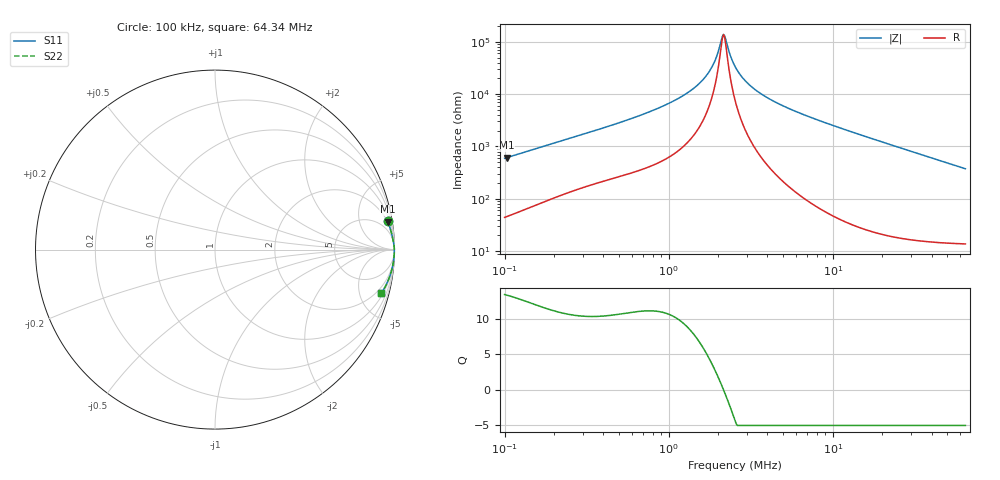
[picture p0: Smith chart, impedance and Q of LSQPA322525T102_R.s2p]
! LSQPA322525T102_R  S-PARAMETER MODEL  ( General Type )
! Model Generated by TAIYO YUDEN Corporation (http://www.ty-top.com)
! Version 1.0
! TAIYO YUDEN Control No. 111018NG25SB-FKC
! Copyright(c) 2011 TAIYO YUDEN CO.,LTD. All Rights Reserved.
! Product Description (link to TY-COMPAS)
! https://ds.yuden.co.jp/TYCOMPAS/or/detail?pn=LSQPA322525T102KR&u=M
! Products Name : Inductors
! Characteristics :
!  Inductance : 1000 uH , SRF(min) : 1.6 MHz , DC Resistance(max) : 16.9 Ohm
!  Rated Current : Saturation :100 mA , Temp Rise : 100 mA (40 degC)
!  Case Size : 3.2 x 2.5 / 0.126 x 0.098 [mm/inch] , Thickness : 2.5 / 0.098 [mm/inch]
!  (Conditions: Temperature = 25 degC , DC Bias Current/Voltage = 0A / 0V)
! External Node Assignments :
!  1  o---GGG---o  2
! GND o---------o GND
! Frequency Range : 0.1MHz  -  64.339822MHz  [ 402 STEP ]
# MHz S RI R 50
! Freq[MHz].  S11 Real  S11 Imag  S21 Real  S21 Imag  S12 Real  S12 Imag  S22 Real  S22 Imag
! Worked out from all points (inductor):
!   401 points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, 100 kHz to 64.34 MHz, reference 50 ohm
!   read as one part in series: L = 932 uH near 103.3 kHz
!   highest Q = 13.3 at 103.3 kHz (marker M1), where L = 941 uH
!   self-resonance near 2.158 MHz
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0.1  0.9612 0.1595  0.0388 -0.1595  0.0388 -0.1595  0.9612 0.1595
0.103286  0.963 0.1549  0.037 -0.1549  0.037 -0.1549  0.963 0.1549
0.295407  0.9909 0.0583  0.0091 -0.0583  0.0091 -0.0583  0.9909 0.0583
0.554941  0.9961 0.0312  0.00387 -0.0312  0.00387 -0.0312  0.9961 0.0312
0.872651  0.998 0.0182  0.00198 -0.0182  0.00198 -0.0182  0.998 0.0182
1.265693  0.9988 0.00995  0.00119 -0.00995  0.00119 -0.00995  0.9988 0.00995
1.613044  0.9991 0.00528  0.000907 -0.00528  0.000907 -0.00528  0.9991 0.00528
1.748849  0.9992 0.0038  0.000842 -0.0038  0.000842 -0.0038  0.9992 0.0038
1.86568  0.9992 0.00263  0.000798 -0.00263  0.000798 -0.00263  0.9992 0.00263
1.958397  0.9992 0.00176  0.00077 -0.00176  0.00077 -0.00176  0.9992 0.00176
2.089227  0.9993 0.000603  0.000739 -0.000603  0.000739 -0.000603  0.9993 0.000603
2.157883  0.9993 2.51e-05  0.000725 -2.51e-05  0.000725 -2.51e-05  0.9993 2.51e-05
2.228796  0.9993 -0.000553  0.000713 0.000553  0.000713 0.000553  0.9993 -0.000553
2.377689  0.9993 -0.00171  0.000694 0.00171  0.000694 0.00171  0.9993 -0.00171
2.53653  0.9993 -0.00288  0.000681 0.00288  0.000681 0.00288  0.9993 -0.00288
2.705981  0.9993 -0.00406  0.000672 0.00406  0.000672 0.00406  0.9993 -0.00406
2.933801  0.9993 -0.00556  0.00067 0.00556  0.00067 0.00556  0.9993 -0.00556
3.619981  0.9993 -0.00965  0.000703 0.00965  0.000703 0.00965  0.9993 -0.00965
4.921632  0.9991 -0.0165  0.000872 0.0165  0.000872 0.0165  0.9991 -0.0165
7.493079  0.9985 -0.0285  0.00146 0.0285  0.00146 0.0285  0.9985 -0.0285
22.13506  0.9902 -0.09  0.00978 0.09  0.00978 0.09  0.9902 -0.09
64.33982  0.9258 -0.2444  0.0742 0.2444  0.0742 0.2444  0.9258 -0.2444
